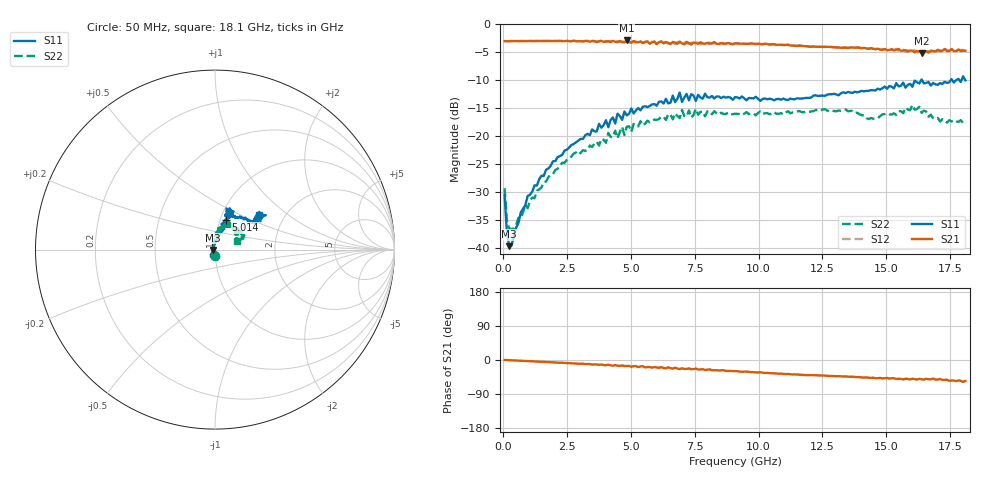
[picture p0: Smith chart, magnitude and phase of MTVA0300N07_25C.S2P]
! Network Analyzer HP8720D.06.14 Serial No. US36140669
! 27 Jun 2005  12:01:14
! Frequency  S11  S21  S12  S22
# HZ  S  DB R 50
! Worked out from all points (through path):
!   201 points, 50 MHz to 18.1 GHz, reference 50 ohm
!   highest |S21| = -2.93 dB at 4.833 GHz (marker M1); lowest = -5.2 dB at 16.39 GHz (marker M2)
!   group delay of S21, straight-line fit = 8.73 ps
!   lowest |S11| = -39.6 dB at 230.5 MHz (marker M3), VSWR 1.02, Z = 49 - j0.238 ohm
!   |S11| at or under -10 dB: start of sweep to 16.37 GHz; 16.4 GHz to 17.53 GHz (1.132 GHz wide, 6.67 % of centre); 17.58 GHz to 17.74 GHz (154.7 MHz wide, 0.876 % of centre)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
!   |S22| runs from -36.6 to -14.4 dB; largest |S21 - S12| = 0.036
!   S11 on the Smith chart (normalised r, x): 50 MHz: 0.98, -0.06; 5.014 GHz: 1.06, +0.36; 18.1 GHz: 1.49, +0.64
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5e7  -30.57 -103.5  -3.04 0.0  -3.05 0.4  -29.29 -89.1
1.4025e8  -37.27 -136.8  -3.08 -0.3  -3.06 -0.2  -35.10 -141.4
2.305e8  -39.63 -166.5  -3.05 -0.5  -3.05 -0.5  -36.50 -164.8
1.22325e9  -28.78 93.8  -3.03 -3.8  -3.04 -3.7  -31.08 109.1
2.30625e9  -23.35 76.0  -3.04 -7.3  -3.03 -7.4  -24.75 91.7
3.1185e9  -20.50 73.7  -3.10 -9.7  -3.11 -10.1  -22.51 88.2
4.65275e9  -17.09 65.9  -3.26 -14.4  -3.09 -15.8  -18.33 81.9
4.743e9  -15.61 68.7  -3.29 -16.0  -3.21 -14.9  -19.79 77.8
4.83325e9  -16.29 73.9  -2.93 -15.7  -3.17 -16.5  -18.33 71.3
5.01375e9  -15.05 70.3  -3.33 -17.7  -3.33 -16.2  -19.23 73.6
6.09675e9  -13.87 67.6  -3.24 -20.7  -3.16 -20.3  -16.94 68.7
6.7285e9  -13.94 73.7  -3.32 -20.2  -3.58 -21.2  -15.93 61.9
6.909e9  -12.22 70.5  -3.13 -24.0  -3.26 -22.1  -16.80 61.6
6.99925e9  -13.90 70.4  -3.44 -21.9  -3.58 -24.0  -15.34 62.4
7.17975e9  -12.47 74.6  -3.18 -23.6  -3.46 -22.3  -16.54 57.0
7.54075e9  -13.71 66.4  -3.41 -22.6  -3.28 -25.5  -15.13 64.5
9.075e9  -13.04 68.0  -3.46 -29.4  -3.43 -29.5  -15.99 51.0
1.21435e10  -12.78 52.7  -4.02 -40.0  -3.98 -40.1  -15.54 44.2
1.512175e10  -11.05 33.4  -4.64 -49.0  -4.45 -48.5  -16.11 37.7
1.602425e10  -11.20 36.8  -4.75 -49.5  -5.01 -51.8  -14.44 30.1
1.638525e10  -9.89 34.6  -5.16 -50.9  -4.82 -50.2  -15.84 24.7
1.81e10  -10.05 38.4  -4.77 -55.4  -4.94 -56.3  -17.44 22.2
